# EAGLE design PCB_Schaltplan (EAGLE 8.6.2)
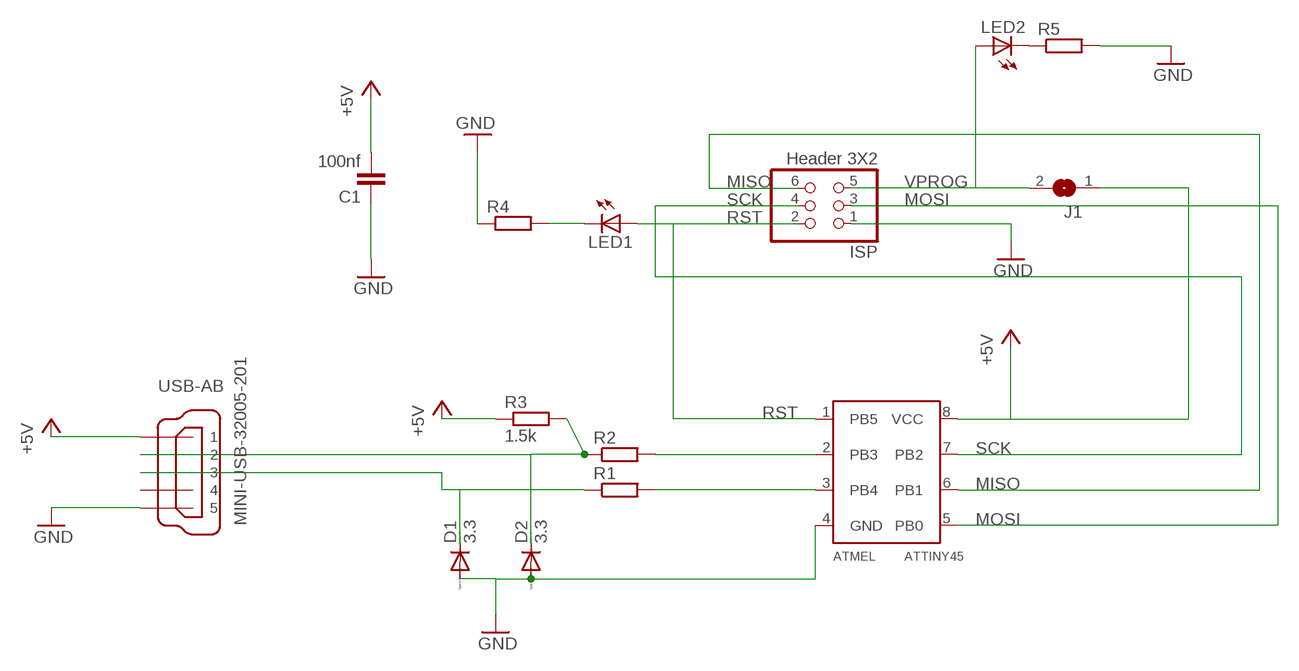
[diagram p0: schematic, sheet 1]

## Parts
ATMEL  ATTINY45  [SOIC8]
C1  100nf  C-EUC1206  [C1206]
D1  3.3  DIODE-MINIMELF  [MINIMELF]
D2  3.3  DIODE-MINIMELF  [MINIMELF]
ISP  Header 3X2  PINHD-2X3SMT  [2X03_SMT]
J1  SJW  [SJW]
LED1  LEDSMT1206  [1206]
LED2  LEDSMT1206  [1206]
R1  R-EU_R1206  [R1206]
R2  R-EU_R1206  [R1206]
R3  1.5k  R-EU_R1206  [R1206]
R4  R-EU_R1206  [R1206]
R5  R-EU_R1206  [R1206]
USB-AB  MINI-USB-32005-201  [32005-201]

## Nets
+5V: ATMEL.8(VCC) C1.2 J1.1 R3.1 USB-AB.1
GND: ATMEL.4(GND) C1.1 D1.A D2.A ISP.1 R4.1 R5.2 USB-AB.5
MISO: ATMEL.6(PB1) ISP.6
MOSI: ATMEL.5(PB0) ISP.3
N$1: ATMEL.2(PB3) R2.2
N$2: ATMEL.3(PB4) R1.2
N$3: LED2.C R5.1
N$4: LED1.C R4.2
N$5: D2.C R2.1 R3.2 USB-AB.2
N$6: D1.C R1.1 USB-AB.3
RST: ATMEL.1(PB5) ISP.2 LED1.A
SCK: ATMEL.7(PB2) ISP.4
VPROG: ISP.5 J1.2 LED2.A
Unconnected: USB-AB.4

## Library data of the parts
ATMEL = attiny45:ATTINY45
C1 = rcl:C-EU: CAPACITOR, European symbol
D1 D2 = diode:DIODE-: DIODE
ISP = pinhead+:PINHD-2X3: PIN HEADER
J1 = jumper:SJ: SMD solder JUMPER
LED1 LED2 = led:LED: LED
R1-R5 = rcl:R-EU_: RESISTOR, European symbol
USB-AB = con-cypressindustries:MINI-USB-: MINI USB-B Conector Source: www.cypressindustries.com; OC_FARNELL: unknown; OC_NEWARK: unknown

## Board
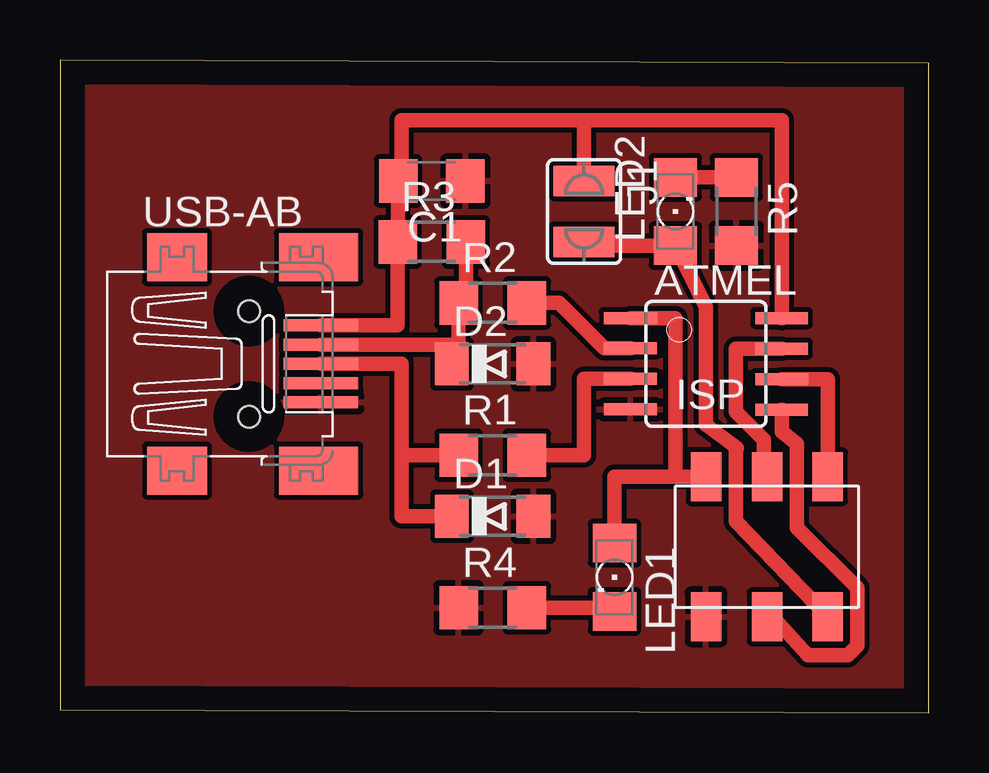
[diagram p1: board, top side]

Size 36.22 x 27.19 mm. Coordinates in mm from the lower left corner, seen from the top.
Outline: 0,0.13 36.22,0 36.22,27.06 0,27.19 0,0.13
Copper layers (1*16): Top 0.035mm / dielectric 1.5mm / Bottom 0.035mm
Design rules "default *": minimum track width 10mil, minimum drill 24mil, track to track 8mil, track to pad 8mil, pad to pad 8mil, via to via 8mil, smd to smd 8mil, copper to edge 40mil, drill to drill 8mil, minimum pad ring 10mil, minimum via ring 8mil, stop-mask expansion 4mil, vias tented up to drill 0mil, thermal gap 10mil

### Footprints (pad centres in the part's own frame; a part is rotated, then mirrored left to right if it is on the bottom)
SOIC8 = smd 0.5 x 2.2: 1 -1.905,-3.154; 2 -0.645,-3.154; 3 0.625,-3.154; 4 1.895,-3.154; 5 1.905,3.154; 6 0.635,3.154; 7 -0.635,3.154; 8 -1.905,3.154
C1206 = smd 1.6 x 1.8: 1 -1.4,0; 2 1.4,0
MINIMELF = smd 1.4 x 1.8: A 1.7,0; C -1.7,0
2X03_SMT = smd 1.27 x 2.032: 1 -2.54,-2.921; 2 -2.54,2.921; 3 0,-2.921; 4 0,2.921; 5 2.54,-2.921; 6 2.54,2.921
SJW = smd 1.27 x 2.54: 1 -1.27,0; 2 1.27,0
1206 = smd 1.6 x 1.803: A -1.422,0; C 1.422,0
R1206 = smd 1.6 x 1.803: 1 -1.422,0; 2 1.422,0
32005-201 = smd 3.1 x 0.5: 1 3,1.6; 2 3,0.8; 3 3,0; 4 3,-0.8; 5 3,-1.6 | smd 2.5 x 2: M1 -3,-4.45; M2 -3,4.45 | smd 3.3 x 2: M3 2.9,4.45; M4 2.9,-4.45 | hole 0.9: 0,2.2; 0,-2.2

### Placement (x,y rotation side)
ATMEL  26.93,14.53 270 top
C1  15.5,22.15 180 top
D1  18.04,8.18 0 top
D2  18.04,14.53 0 top
ISP  29.47,6.91 0 top
J1  21.85,20.88 270 top
LED1  23.12,5.64 270 top
LED2  25.66,20.88 90 top
R1  18.04,10.72 0 top
R2  18.04,17.07 0 top
R3  15.5,19.61 0 top
R4  18.04,4.37 0 top
R5  28.2,20.88 270 top
USB-AB  7.88,14.53 0 top

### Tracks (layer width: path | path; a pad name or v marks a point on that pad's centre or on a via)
+5V
  Top 0.61: USB-AB.1 14.08,16.13 R3.1 14.1,19.61 C1.2 14.23,22.15 14.23,24.69 21.85,24.69 | 21.85,24.69 J1.1 | 21.85,24.69 30.08,24.69 ATMEL.8
GND
  pour Top: -4.82,33.58 45.98,33.58 45.98,-4.52 -4.82,-4.52
MISO
  Top 0.61: ISP.6 32.01,13.9 ATMEL.6
MOSI
  Top 0.61: ATMEL.5 30.08,11.71 30.71,11.2 30.71,7.71 33.24,5.2 33.24,2.79 32.83,2.4 31.19,2.4 29.71,3.99 ISP.3
N$1
  Top 0.61: 19.59,16.95 R2.2 20.81,17.07 22.71,15.18 ATMEL.2
N$2
  Top 0.61: ATMEL.3 21.85,13.91 21.85,10.72 R1.2
N$3
  Top 0.61: LED2.C R5.1
N$4
  Top 0.61: LED1.C 23.12,4.37 R4.2
N$5
  Top 0.61: USB-AB.2 16.34,15.33 D2.C 16.62,14.53 R2.1 16.92,17.07 R3.2
N$6
  Top 0.61: USB-AB.3 14.23,14.53 14.23,10.72 | 14.23,10.72 14.23,8.18 D1.C | R1.1 14.23,10.72
RST
  Top 0.61: ATMEL.1 25.66,16.44 25.66,9.83 | 25.66,9.83 ISP.2 | 25.66,9.83 23.12,9.83 LED1.A
SCK
  Top 0.61: ATMEL.7 28.18,15.17 | 28.18,15.17 | 28.18,15.17 28.18,12.53 29.35,11.36 | 29.35,11.36 | 29.35,11.36 29.35,9.83 ISP.4
VPROG
  Top 0.61: J1.2 21.85,19.46 LED2.A 26.93,16.92 26.93,11.99 28.07,11.15 28.22,11.02 28.18,11.03 28.18,7.97 ISP.5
